FUNCTION_BLOCK FB_SAFE_CONTROL
VAR_INPUT
	ManErrAck										:	BOOL;

	// CONTROL
	Run										AT%Q*	:	BOOL := TRUE;
	ErrAck									AT%Q*	:	BOOL;
	Restart									AT%Q*	:	BOOL;

END_VAR
VAR_OUTPUT
	ComErr									AT%I*	:	BOOL;
	OtherErr								AT%I*	:	BOOL;
	InRun									AT%I*	:	BOOL;

END_VAR
VAR
	_ton20ms										:	TON;
END_VAR

_ton20ms(IN:= ManErrAck, PT:= T#20MS, Q=> , ET=> );

IF _ton20ms.Q THEN 
	ManErrAck := FALSE;
END_IF

IF NOT ManErrAck
THEN 
	IF OtherErr OR ComErr 
	THEN  
		ErrAck := TRUE;
	ELSE
		ErrAck := FALSE;
	END_IF
ELSE
	ErrAck := ManErrAck;
END_IF

END_FUNCTION_BLOCK
